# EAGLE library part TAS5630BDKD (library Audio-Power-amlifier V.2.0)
300W STEREO / 600W MONO PurePath ? HD ANALOG-INPUT POWER STAGE CW07/2009
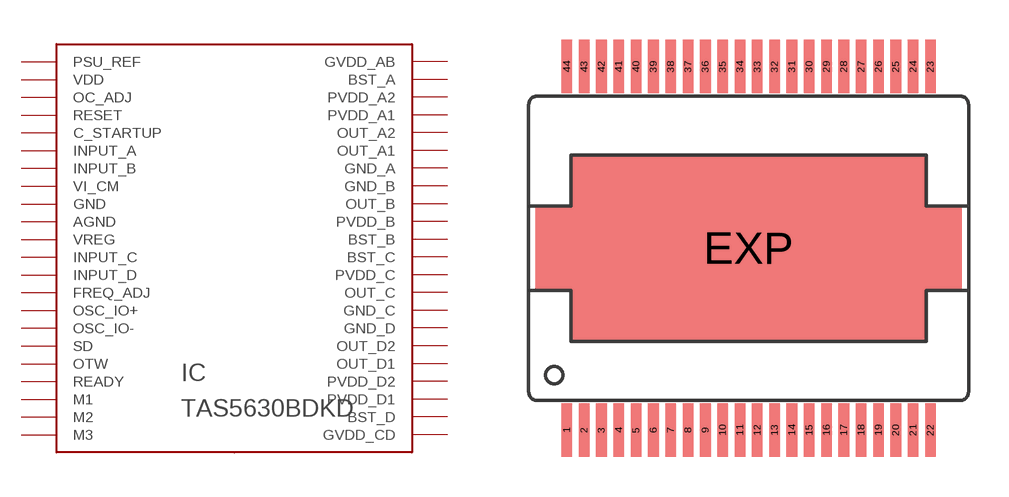
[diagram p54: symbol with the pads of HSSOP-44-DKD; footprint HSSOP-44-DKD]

Designator prefix IC

## TAS5630BDKD  [HSSOP-44-DKD]
1  PSU_REF
2  VDD
3  OC_ADJ
4  RESET
5  C_STARTUP
6  INPUT_A
7  INPUT_B
8  VI_CM
9  GND
10  AGND
11  VREG
12  INPUT_C
13  INPUT_D
14  FREQ_ADJ
15  OSC_IO+
16  OSC_IO-
17  SD
18  OTW
19  READY
20  M1
21  M2
22  M3
23  GVDD_CD
24  BST_D
25  PVDD_D1
26  PVDD_D2
27  OUT_D1
28  OUT_D2
29  GND_D
30  GND_C
31  OUT_C
32  PVDD_C
33  BST_C
34  BST_B
35  PVDD_B
36  OUT_B
37  GND_B
38  GND_A
39  OUT_A1
40  OUT_A2
41  PVDD_A1
42  PVDD_A2
43  BST_A
44  GVDD_AB

## Footprint HSSOP-44-DKD (pad centres in mm)
HSSOP44-DKD. www.ti.com/audio
smd 0.4 x 2: 1 -6.825,-6.825; 2 -6.175,-6.825; 3 -5.525,-6.825; 4 -4.875,-6.825; 5 -4.225,-6.825; 6 -3.575,-6.825; 7 -2.925,-6.825; 8 -2.275,-6.825; 9 -1.625,-6.825; 10 -0.975,-6.825; 11 -0.325,-6.825; 12 0.325,-6.825; 13 0.975,-6.825; 14 1.625,-6.825; 15 2.275,-6.825; 16 2.925,-6.825; 17 3.575,-6.825; 18 4.225,-6.825; 19 4.875,-6.825; 20 5.525,-6.825; 21 6.175,-6.825; 22 6.825,-6.825; 23 6.825,6.825; 24 6.175,6.825; 25 5.525,6.825; 26 4.875,6.825; 27 4.225,6.825; 28 3.575,6.825; 29 2.925,6.825; 30 2.275,6.825; 31 1.625,6.825; 32 0.975,6.825; 33 0.325,6.825; 34 -0.325,6.825; 35 -0.975,6.825; 36 -1.625,6.825; 37 -2.275,6.825; 38 -2.925,6.825; 39 -3.575,6.825; 40 -4.225,6.825; 41 -4.875,6.825; 42 -5.525,6.825; 43 -6.175,6.825; 44 -6.825,6.825
smd 13.3 x 7: EXP 0,0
